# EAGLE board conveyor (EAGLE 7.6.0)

Size 73.58 x 88.79 mm. Coordinates in mm from the lower left corner, seen from the top.
Outline: 0,0 56.82,0 56.82,53.33 0,53.33 0,0
Copper layers (1*16): Top 0.035mm / dielectric 1.5mm / Bottom 0.035mm
Design rules "default": minimum track width 10mil, minimum drill 24mil, track to track 8mil, track to pad 8mil, pad to pad 8mil, via to via 8mil, smd to smd 8mil, copper to edge 40mil, drill to drill 8mil, minimum pad ring 10mil, minimum via ring 8mil, stop-mask expansion 4mil, vias tented up to drill 0mil, thermal gap 10mil

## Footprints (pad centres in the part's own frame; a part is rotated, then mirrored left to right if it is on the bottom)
LED5MM = drill 0.813 octagon: A -1.27,0; K 1.27,0
D-7.5 = drill 0.813 long: A 3.81,0; C -3.81,0
2P-2.54-65/35MIL = drill 0.889 pad 1.651 square: 1 0,1.27 | drill 0.889 pad 1.651: 2 0,-1.27
PHOTORESISTOR-2.54 = drill 1 pad 1.5: P$1 -1.27,0; P$2 1.27,0
TO220 = drill 1.118 long: 1 -2.54,-6.35; 2 0,-6.35; 3 2.54,-6.35 | hole 3.302: 0,11.176
0207/10 = drill 0.813 octagon: 1 -5.08,0; 2 5.08,0
ARDUINO_UNO = drill 1.016 pad 1.88: 0 63.5,50.8; 1 60.96,50.8; 2 58.42,50.8; 3 55.88,50.8; 3.3V 35.56,2.54; 4 53.34,50.8; 5 50.8,50.8; 5V 38.1,2.54; 6 48.26,50.8; 7 45.72,50.8; 8 41.656,50.8; 9 39.116,50.8; 10 36.576,50.8; 11 34.036,50.8; 12 31.496,50.8; 13 28.956,50.8; A0 50.8,2.54; A1 53.34,2.54; A2 55.88,2.54; A3 58.42,2.54; A4 60.96,2.54; A5 63.5,2.54; AREF 23.876,50.8; GND 26.416,50.8; GND. 43.18,2.54; GND.. 40.64,2.54; I/OREF 30.48,2.54; N/C 27.94,2.54; RESET 33.02,2.54; SCL 18.796,50.8; SDA 21.336,50.8; VIN 45.72,2.54 | hole 3.2: 66.04,7.62; 66.04,35.56; 15.24,50.8; 13.97,2.54

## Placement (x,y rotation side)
D1  [LED5MM]  5,10.08 0 top
D2  [D-7.5]  not placed on the board
M1  [2P-2.54-65/35MIL]  5,60.88 0 top
P1  24V  [2P-2.54-65/35MIL]  5,73.58 0 top
Q1  [PHOTORESISTOR-2.54]  5,48.18 0 top
Q2  [TO220]  5,86.28 0 top
R2  10k‎Ω  [0207/10]  5,22.78 0 top
R3  1k‎Ω  [0207/10]  not placed on the board
U1  [ARDUINO_UNO]  5,35.48 0 top

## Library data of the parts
D1 D2 M1 P1 Q1 Q2 R2 R3 U1 = AUTODESK_CIRCUITS_BREADBOARD

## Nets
N$1: Q1.P$2 U1.5V
N$2: D1.K Q1.P$1 R2.1 R2.2 U1.A0 U1.GND..
N$3: D2.A M1.2 P1.2
N$4: D1.A R3.2
N$5: D2.C M1.1 Q2.3
N$6: Q2.2 R3.1 U1.5
N$7: P1.1 Q2.1

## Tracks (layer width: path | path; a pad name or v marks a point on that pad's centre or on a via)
N$1  (1 unrouted)
N$2  (5 unrouted)
N$3  (2 unrouted)
N$4  (1 unrouted)
N$5  (2 unrouted)
N$6  (2 unrouted)
N$7  (1 unrouted)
